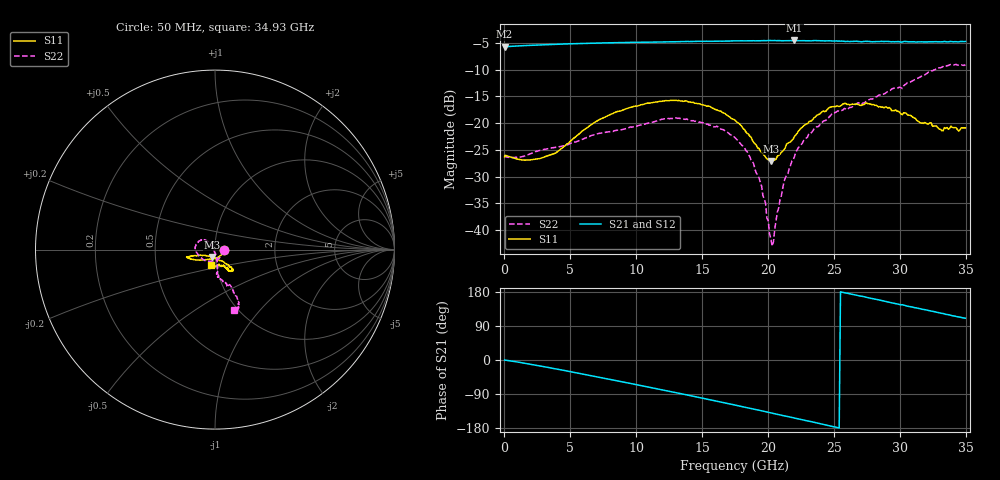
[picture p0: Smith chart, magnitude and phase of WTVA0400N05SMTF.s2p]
! 50 ohm 2-Port S-parameters measured by Modelithics Inc support@modelithics.com  Tampa, FL USA 813-866-6335 (February 2024)
! Smiths Interconnect,  4dB P/N: WTVA0400N05SMTF, Temperature: -25 C
! Board: 10 mil Rogers 4350B, Mounting Pad Dimensions: Length: 15 mils, Width: 25 mils, Gap: 40 mils.
# Hz S RI R 50
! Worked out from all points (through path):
!   352 points, 50 MHz to 34.93 GHz, reference 50 ohm
!   highest |S21| = -4.51 dB at 21.99 GHz (marker M1); lowest = -5.7 dB at 50 MHz (marker M2)
!   group delay of S21, straight-line fit = 20.3 ps
!   lowest |S11| = -27.1 dB at 20.2 GHz (marker M3), VSWR 1.09, Z = 48.3 - j3.99 ohm
!   |S11| at or under -10 dB: start of sweep to end of sweep
!   |S22| runs from -43.0 to -9.0 dB; largest |S21 - S12| = 0.0064
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5e7  0.0484 -0.00133  0.52 -0.00106  0.5193 -0.00138  0.0501 -0.00134
2.8865e9  0.00737 -0.0468  0.5179 -0.1561  0.5171 -0.1559  0.0189 -0.0531
5.8715e9  -0.0606 -0.0572  0.4488 -0.3311  0.4479 -0.3311  -0.0258 -0.0652
8.4585e9  -0.1134 -0.0569  0.3321 -0.4592  0.3308 -0.4592  -0.0647 -0.0557
1.1742e10  -0.1536 -0.045  0.1279 -0.5605  0.1263 -0.5602  -0.1063 -0.0114
1.48265e10  -0.1467 -0.0396  -0.0945 -0.576  -0.0955 -0.5751  -0.0938 0.0423
1.7513e10  -0.1003 -0.0336  -0.2871 -0.5153  -0.2883 -0.5137  -0.0508 0.0522
1.84085e10  -0.0733 -0.0323  -0.3465 -0.4792  -0.347 -0.4781  -0.0354 0.041
1.9304e10  -0.0462 -0.0351  -0.3993 -0.4354  -0.4005 -0.4334  -0.0219 0.0216
1.98015e10  -0.0297 -0.0376  -0.4302 -0.4087  -0.4303 -0.4077  -0.0134 0.0117
1.9901e10  -0.026 -0.0386  -0.4344 -0.4029  -0.4346 -0.4018  -0.0111 0.00663
2.01995e10  -0.0159 -0.0413  -0.4518 -0.3863  -0.4521 -0.3848  -0.00829 -0.000196
2.0299e10  -0.0121 -0.0425  -0.4569 -0.3795  -0.4575 -0.3776  -0.00658 -0.00257
2.03985e10  -0.00896 -0.0441  -0.4623 -0.3737  -0.463 -0.3717  -0.00504 -0.00589
2.0697e10  0.00181 -0.0493  -0.4764 -0.3533  -0.4772 -0.3509  -0.00282 -0.0145
2.11945e10  0.0166 -0.054  -0.4961 -0.3202  -0.4965 -0.3182  0.0033 -0.0282
2.19905e10  0.0381 -0.0648  -0.5314 -0.2676  -0.5315 -0.2655  0.0109 -0.0475
2.33835e10  0.071 -0.0822  -0.5681 -0.1676  -0.5678 -0.1659  0.014 -0.0838
2.57715e10  0.1014 -0.1144  -0.5825 0.0256  -0.5817 0.027  0.0112 -0.1371
2.91545e10  0.0759 -0.1179  -0.5151 0.2697  -0.5131 0.272  0.0624 -0.1907
3.31345e10  0.0181 -0.0833  -0.3148 0.4841  -0.311 0.4857  0.1335 -0.3067
3.49255e10  -0.0222 -0.0876  -0.2021 0.5461  -0.1968 0.5473  0.1076 -0.3355
